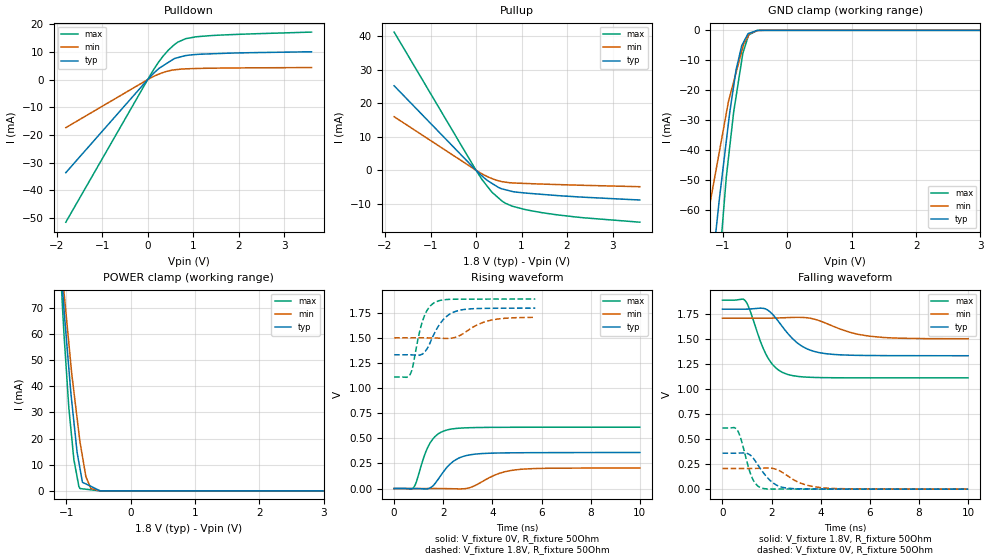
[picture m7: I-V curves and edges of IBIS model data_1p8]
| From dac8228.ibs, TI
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|   data_1p8 Model
[Model]   data_1p8
Model_type   I/O
Polarity   Non-Inverting
Enable   Active-Low
Vinl = 0.3
Vinh = 1.5
Vmeas = 0.9
Vref = 0.9
Cref = 10pF
Rref = 50
|   typ   min   max
|   (nom PVT)   (Fast PVT)   (slow PVT)
|C_comp from frequency method(F=50MHz)
C_comp   1.085e-11   9.210e-12   1.238e-11
|ON state : BUFFER OUTPUT TURNED HIGH
|C_comp   1.085e-11   9.210e-12   1.238e-11
|OFF state: BUFFER IN HIGH IMPEDANCE
|C_comp   1.058e-11   8.952e-12   1.206e-11
|C_comp from L-C Tank method(L=1nH)
|Average
|C_comp   9.843e-12   8.5715e-12  1.1045e-11
|ON state : BUFFER OUTPUT TURNED HIGH
|Resonant Frequency(Hz)   1.6e9   1.71e9   1.51e9
|C_comp   9.904e-12   8.671e-12   1.112e-11
|OFF state: BUFFER IN HIGH IMPEDANCE
|Resonant Frequency(Hz)   1.61e9   1.73e9   1.52e9
|C_comp   9.782e-12   8.472e-12   1.097e-11
| Where nom  PVT is Nominal Process,  1.8V,  33C
|   Fast PVT is Strong Process,   1.89V,  -40C
|   Slow PVT is Weak Process,   1.71V,  113C
[Voltage Range]   1.8   1.71   1.89
|Ambient Temperature   25   105   -40
|Junction Temperature
[Temperature Range]   33   113   -40
[Pullup Reference]   1.8   1.71   1.89
[Pulldown Reference]   0   0   0
[Power Clamp Reference]   1.8   1.71   1.89
[GND Clamp Reference]   0   0   0
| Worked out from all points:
|   slope of the pulldown table from 0 to 0.27 V, typ, clamps not added: 63 ohm
|   slope of the pullup table from 0 to 0.27 V, typ, clamps not added: 83.7 ohm
|   GND clamp passes 1 mA (typ) near -0.60 V on its own axis
|   POWER clamp passes 1 mA (typ) near -0.56 V on its own axis
|   falling waveform, V_fixture 1.8V, R_fixture 50Ohm: 20-80 % time 1.07ns typ, 1.49ns min, 778ps max; typ from 1.8 V to 1.33 V
|   rising waveform, V_fixture 0V, R_fixture 50Ohm: 20-80 % time 781ps typ, 1.08ns min, 586ps max; typ from 0 V to 0.359 V
|   rising waveform, V_fixture 1.8V, R_fixture 50Ohm: 20-80 % time 671ps typ, 944ps min, 452ps max; typ from 1.33 V to 1.8 V
|   falling waveform, V_fixture 0V, R_fixture 50Ohm: 20-80 % time 692ps typ, 960ps min, 426ps max; typ from 0.36 V to 0 V
[Pulldown]
|   Voltage   I(typ)   I(min)   I(max)
-1.8V     -33.62mA   -17.36mA   -51.51mA
94.5mV    1.679mA    857.6uA    2.685mA
252mV     4.1mA      2.016mA    6.598mA
332.6mV   4.946mA    2.529mA    8.364mA
451.7mV   6.194mA    3.101mA    10.6mA
574.6mV   7.482mA    3.512mA    12.48mA
667.2mV   7.964mA    3.67mA     13.57mA
835.4mV   8.669mA    3.878mA    14.78mA
1.089V    9.099mA    4.018mA    15.5mA
1.784V    9.552mA    4.186mA    16.21mA
3.6V      10.05mA    4.348mA    17.16mA
[GND Clamp]
|   Voltage   I(typ)   I(min)   I(max)
-1.8V     -217.1mA   -140.2mA   -312.5mA
-1.262V   -97.62mA   -64.76mA   -140mA
-1.217V   -88.59mA   -59.47mA   -125.7mA
-1.058V   -56.53mA   -40.62mA   -77.97mA
-952.6mV  -37.5mA    -28.06mA   -49.75mA
-916.6mV  -31.03mA   -23.81mA   -42.75mA
-835.4mV  -18.63mA   -17.2mA    -27.34mA
-797.4mV  -13.17mA   -14.11mA   -22.1mA
-693.6mV  -4.462mA   -5.652mA   -7.799mA
-612mV    -1.105mA   -2.018mA   -2.18mA
-447.9mV  -29.85uA   -62.66uA   -17.6uA
3.6V      0A         0A         0A
[Pullup]
|   Voltage   I(typ)   I(min)   I(max)
-1.8V     25.17mA    15.96mA    41.17mA
0V        0A         0A         0A
136.1mV   -1.761mA   -1.108mA   -2.847mA
332.6mV   -3.755mA   -2.38mA    -6.248mA
574.6mV   -5.556mA   -3.404mA   -9.208mA
797.6mV   -6.326mA   -3.765mA   -10.71mA
1.16V     -6.87mA    -3.97mA    -11.93mA
1.542V    -7.277mA   -4.151mA   -12.82mA
2.362V    -8.026mA   -4.483mA   -14.15mA
3.6V      -8.85mA    -4.899mA   -15.47mA
[POWER Clamp]
|   Voltage   I(typ)   I(min)   I(max)
-1.8V     358mA      304.5mA    426.4mA
-1.132V   102.5mA    100.6mA    102.4mA
-1.033V   68.07mA    74.92mA    58.33mA
-960.1mV  46.27mA    55.98mA    31.26mA
-884.5mV  26.67mA    38.19mA    12.16mA
-833.4mV  14.7mA     27.77mA    5.309mA
-790mV    8.732mA    18.93mA    916.8uA
-750.6mV  3.31mA     13.22mA    803.6uA
-696mV    2.662mA    5.386mA    646.8uA
-619mV    1.749mA    918.7uA    426uA
-470.3mV  197.2nA    12.34uA    3.023nA
3.6V      0A         0A         0A
[Ramp]
R_load = 50
|   typ   min   max
dV/dt_r   0.215662/7.79359e-10   0.123488/1.07653e-09   0.366952/5.85424e-10
dV/dt_f   0.279411/1.06685e-09   0.123695/1.47841e-09   0.466234/7.74647e-10
[Falling Waveform]
V_fixture = 1.8V
V_fixture_min = 1.71V
V_fixture_max = 1.89V
R_fixture = 50Ohm
|   Time   V(typ)   V(min)   V(max)
0s        1.8V       1.71V      1.89V
926ps     1.8V       1.71V      1.884V
1.128ns   1.802V     1.71V      1.782V
1.837ns   1.791V     1.71V      1.319V
2.199ns   1.703V     1.712V     1.207V
2.64ns    1.563V     1.716V     1.149V
3.407ns   1.407V     1.715V     1.121V
4.245ns   1.354V     1.656V     1.115V
5.966ns   1.337V     1.53V      1.113V
10ns      1.334V     1.504V     1.113V
[Rising Waveform]
V_fixture = 0V
V_fixture_min = 0V
V_fixture_max = 0V
R_fixture = 50Ohm
|   Time   V(typ)   V(min)   V(max)
0s        1.583nV    2.419nV    1.294nV
774ps     254.2uV    6.49uV     5.26mV
1.25ns    -3.945mV   87.28uV    341.2mV
1.461ns   5.743mV    150uV      453.6mV
1.786ns   90.31mV    133.3uV    543.7mV
2.189ns   222.3mV    -1.004mV   586.4mV
3.08ns    336mV      8.705mV    606.9mV
4.071ns   353.5mV    131.6mV    610.3mV
4.91ns    356.5mV    185.6mV    611.1mV
10ns      359.4mV    205.8mV    611.6mV
[Rising Waveform]
V_fixture = 1.8V
V_fixture_min = 1.71V
V_fixture_max = 1.89V
R_fixture = 50Ohm
|   Time   V(typ)   V(min)   V(max)
0s        1.334V     1.503V     1.113V
640ps     1.334V     1.503V     1.134V
741ps     1.333V     1.503V     1.199V
962ps     1.328V     1.503V     1.482V
1.173ns   1.345V     1.503V     1.684V
1.633ns   1.545V     1.502V     1.854V
2.087ns   1.707V     1.497V     1.884V
2.632ns   1.776V     1.521V     1.889V
3.844ns   1.798V     1.674V     1.89V
5.745ns   1.799V     1.708V     1.89V
[Falling Waveform]
V_fixture = 0V
V_fixture_min = 0V
V_fixture_max = 0V
R_fixture = 50Ohm
|   Time   V(typ)   V(min)   V(max)
0s        359.6mV    206.7mV    611.6mV
595ps     359.9mV    206.6mV    595.5mV
765ps     361.9mV    206.5mV    490.2mV
1.205ns   323.8mV    207.1mV    114.3mV
1.407ns   255.9mV    208.1mV    38.54mV
1.645ns   170.1mV    210.2mV    7.404mV
2.185ns   42.66mV    198.2mV    1.039mV
2.868ns   5.256mV    97.55mV    1.145mV
4.139ns   1.618mV    12.31mV    293.8uV
10ns      80.42uV    466.3uV    737.8nV
